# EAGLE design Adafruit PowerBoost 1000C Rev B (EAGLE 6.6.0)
COMPANY: ADAFRUIT INDUSTRIES; DRAWN: KTOWN; REV: A
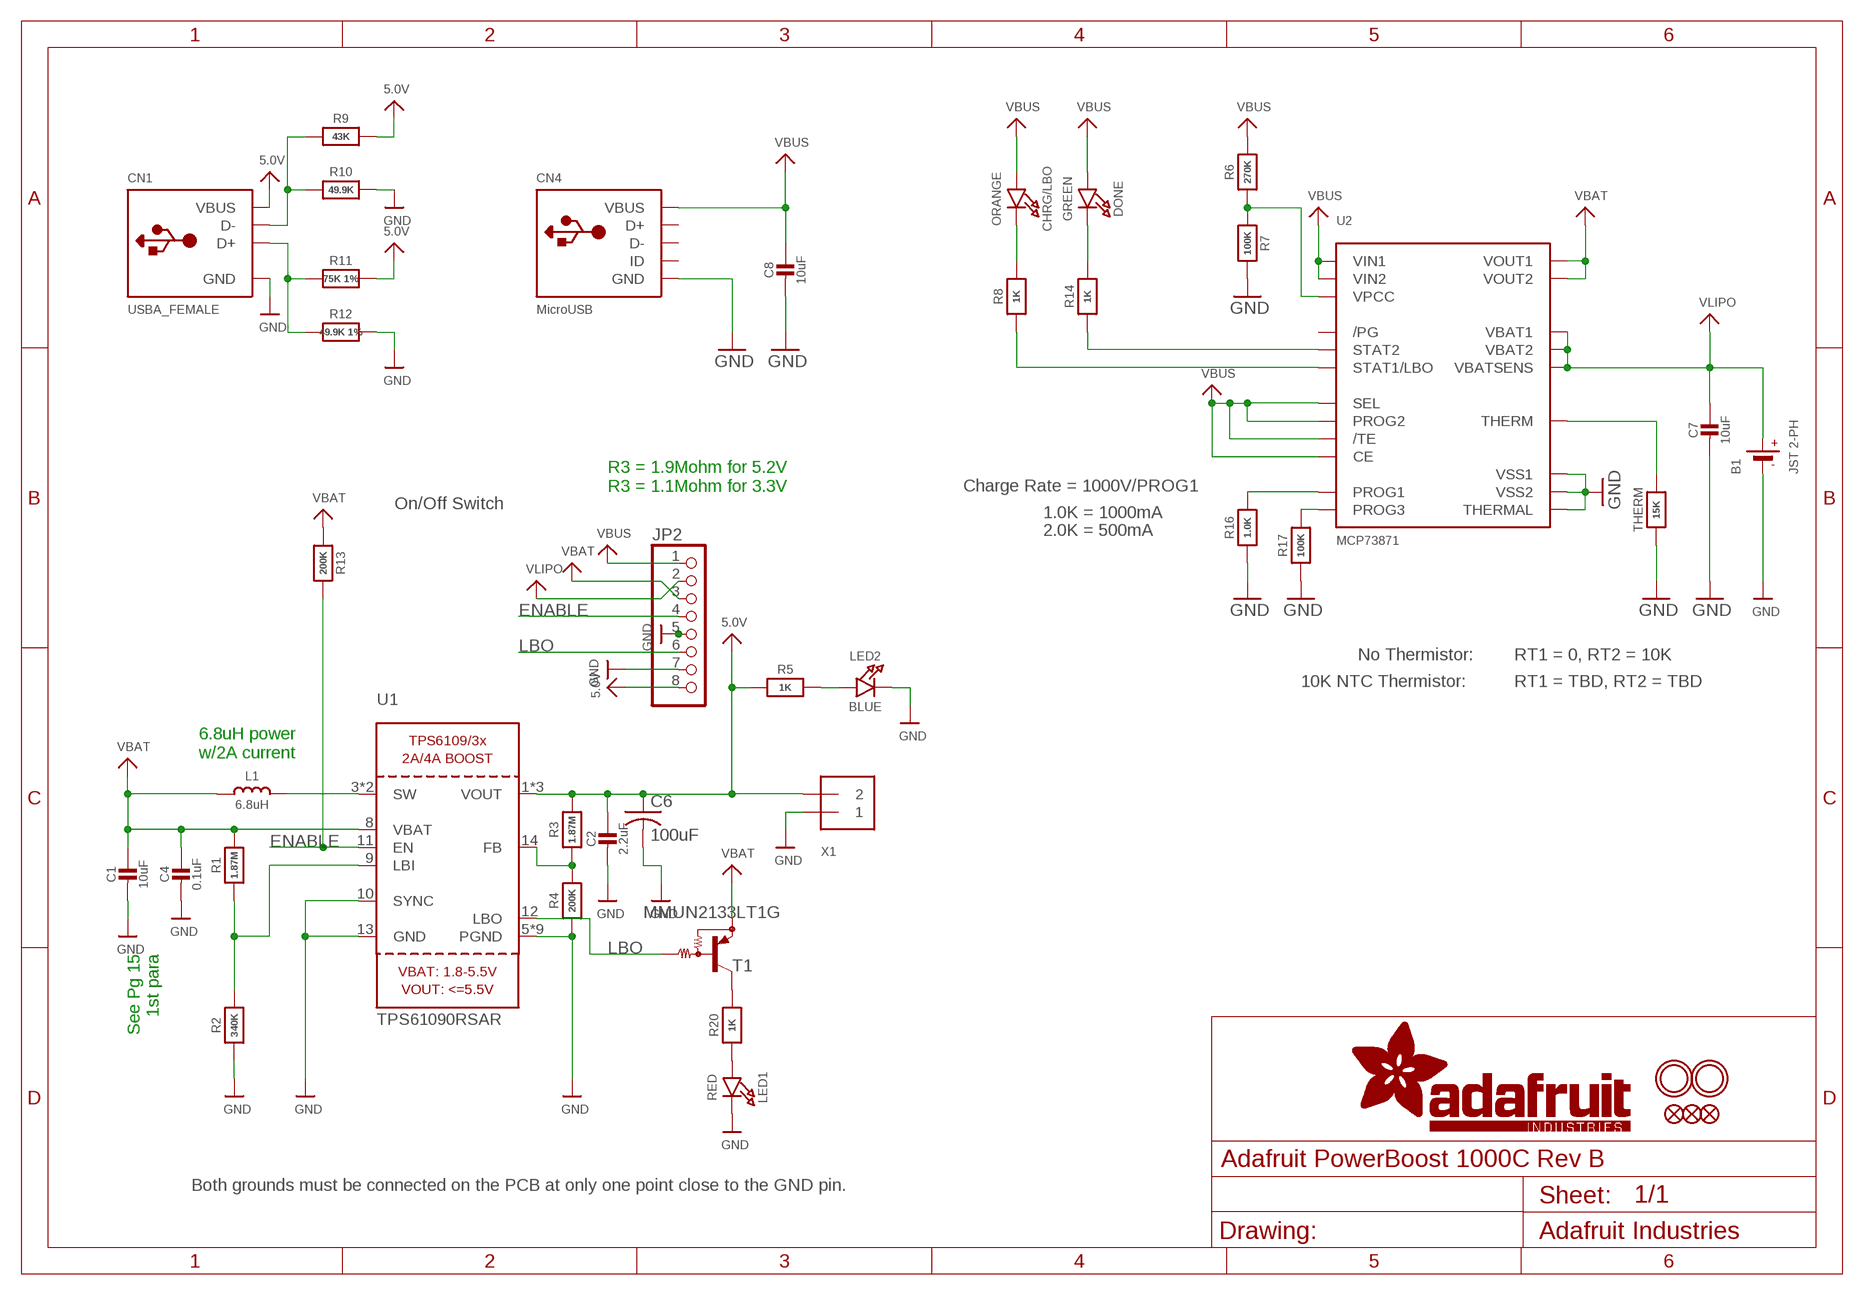
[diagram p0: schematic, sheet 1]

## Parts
B1  JST 2-PH  BATTERY  [JSTPH2]
C1  10uF  CAP_CERAMIC0805-NOOUTLINE  [0805-NO]
C2  2.2uF  CAP_CERAMIC0805-NOOUTLINE  [0805-NO]
C4  0.1uF  CAP_CERAMIC0805_10MGAP  [0805_10MGAP]
C6  100uF  C-USC1210  [C1210]
C7  10uF  CAP_CERAMIC0805-NOOUTLINE  [0805-NO]
C8  10uF  CAP_CERAMIC0805-NOOUTLINE  [0805-NO]
CHRG/LBO  ORANGE  LED0805_NOOUTLINE  [CHIPLED_0805_NOOUTLINE]
CN1  USBA_FEMALE  USB_TYPEAPTHFML  [USB_HOST-PTH]
CN4  MicroUSB  USBMICRO_20329  [4UCONN_20329]
DONE  GREEN  LED0805_NOOUTLINE  [CHIPLED_0805_NOOUTLINE]
FID1  FIDUCIAL""  [FIDUCIAL_1MM]
FID2  FIDUCIAL""  [FIDUCIAL_1MM]
FID3  FIDUCIAL""  [FIDUCIAL_1MM]
JP2  HEADER-1X8ROUND  [1X08_ROUND]
L1  6.8uH  INDUCTORTDK_VLC5045  [INDUCTOR_5X5MM_TDK_VLC5045]
LED1  RED  LED0805_NOOUTLINE  [CHIPLED_0805_NOOUTLINE]
LED2  BLUE  LED0805_NOOUTLINE  [CHIPLED_0805_NOOUTLINE]
R1  1.87M  RESISTOR_0805MP  [_0805MP]
R2  340K  RESISTOR_0805MP  [_0805MP]
R3  1.87M  RESISTOR0805_NOOUTLINE  [0805-NO]
R4  200K  RESISTOR0805_NOOUTLINE  [0805-NO]
R5  1K  RESISTOR0805_NOOUTLINE  [0805-NO]
R6  270K  RESISTOR0805_NOOUTLINE  [0805-NO]
R7  100K  RESISTOR0805_NOOUTLINE  [0805-NO]
R8  1K  RESISTOR0805_NOOUTLINE  [0805-NO]
R9  43K  RESISTOR0805_NOOUTLINE  [0805-NO]
R10  49.9K  RESISTOR0805_NOOUTLINE  [0805-NO]
R11  75K 1%  RESISTOR0805_NOOUTLINE  [0805-NO]
R12  49.9K 1%  RESISTOR0805_NOOUTLINE  [0805-NO]
R13  200K  RESISTOR0805_NOOUTLINE  [0805-NO]
R14  1K  RESISTOR0805_NOOUTLINE  [0805-NO]
R16  1.0K  RESISTOR0805_NOOUTLINE  [0805-NO]
R17  100K  RESISTOR0805_NOOUTLINE  [0805-NO]
R20  1K  RESISTOR0805_NOOUTLINE  [0805-NO]
T1  MMUN2133LT1G  MUN2114T1-PNP_DRIVER-SC59-BEC  [SC59-BEC]
THERM  15K  RESISTOR0805_NOOUTLINE  [0805-NO]
U1  TPS61090RSAR  VREG_TPS6103X  [PVQFN-16]
U2  MCP73871  [QFN20_4MM]
U$10  MOUNTINGHOLE2.5  [MOUNTINGHOLE_2.5_PLATED]
U$11  MOUNTINGHOLE2.5  [MOUNTINGHOLE_2.5_PLATED]
X1  TERMBLOCK_1X2  [TERMBLOCK_1X2-3.5MM]

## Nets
5.0V: C2.1 C6.1 CN1.VBUS JP2.8 R3.2 R5.1 R9.2 R11.2 U1.1(VOUT) U1.15(VOUT) U1.16(VOUT) X1.2
D+: CN1.D+ R11.1 R12.1
D-: CN1.D- R9.1 R10.1
ENABLE: JP2.4 R13.2 U1.11(EN)
GND: B1.1(-) C1.2 C2.2 C4.2 C6.2 C7.2 C8.2 CN1.GND CN4.BASE@1(GND) CN4.BASE@2(GND) CN4.GND CN4.SPRT@1(GND) CN4.SPRT@2(GND) CN4.SPRT@3(GND) CN4.SPRT@4(GND) JP2.5 JP2.7 LED1.C LED2.C R2.1 R4.1 R7.2 R10.2 R12.2 R16.1 R17.1 THERM.1 U1.5(PGND) U1.6(PGND) U1.7(PGND) U1.10(SYNC) U1.13(GND) U1.P$18(PGND) U1.P$19(PGND) U1.P$20(PGND) U1.P$21(PGND) U1.P$22(PGND) U1.THERMAL(PGND) U2.P$10(VSS1) U2.P$11(VSS2) U2.P$21(THERMAL) X1.1
LBO: JP2.6 T1.B U1.12(LBO)
N$1: L1.P$2 U1.3(SW) U1.4(SW)
N$2: LED1.A R20.1
N$3: R1.1 R2.2 U1.9(LBI)
N$4: LED2.A R5.2
N$5: R3.1 R4.2 U1.14(FB)
N$6: R20.2 T1.C
N$7: R6.1 R7.1 U2.P$2(VPCC)
N$8: DONE.C R14.2
N$9: R14.1 U2.P$7(STAT2)
N$10: THERM.2 U2.P$5(THERM)
N$11: R8.1 U2.P$8(STAT1/LBO)
N$12: CHRG/LBO.C R8.2
N$13: R17.2 U2.P$12(PROG3)
N$16: R16.2 U2.P$13(PROG1)
VBAT: C1.1 C4.1 JP2.3 L1.P$1 R1.2 R13.1 T1.E U1.8(VBAT) U2.P$1(VOUT1) U2.P$20(VOUT2)
VBUS: C8.1 CHRG/LBO.A CN4.VBUS DONE.A JP2.1 R6.2 U2.P$3(SEL) U2.P$4(PROG2) U2.P$9(/TE) U2.P$17(CE) U2.P$18(VIN1) U2.P$19(VIN2)
VLIPO: B1.2(+) C7.1 JP2.2 U2.P$14(VBAT1) U2.P$15(VBAT2) U2.P$16(VBATSENS)
Unconnected: CN4.D+ CN4.D- CN4.ID U2.P$6(/PG)

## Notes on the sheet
- R3 = 1.9Mohm for 5.2V
  R3 = 1.1Mohm for 3.3V
- Charge Rate = 1000V/PROG1
- On/Off Switch
- 1.0K = 1000mA
- 2.0K = 500mA
- No Thermistor: | RT1 = 0, RT2 = 10K
- 10K NTC Thermistor: | RT1 = TBD, RT2 = TBD
- 6.8uH power
  w/2A current
- See Pg 15
  1st para
- Both grounds must be connected on the PCB at only one point close to the GND pin.

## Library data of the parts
B1 = microbuilder:BATTERY: CR1220 SMT - Digikey: 3001K-ND
C1 C2 C4 C7 C8 = microbuilder:CAP_CERAMIC: Ceramic Capacitors
C6 = rcl:C-US: CAPACITOR, American symbol
CHRG/LBO DONE LED1 LED2 = microbuilder:LED: LED
CN1 = microbuilder:USB_TYPEA: USB - Type A Connectors Male types stick out and are inserted into a PC or matching females parts (these are the connectors used on USB Memory Sticks, etc.). Female parts are generally used for USB Host and accept a male-type connector. SMT - 4UCON: 10017 PTHFML - Digikey: 609-1045-ND, 4UCon: 05241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
CN4 = microbuilder:USB: USB Connectors USBMINIB - Surface Mount Female Mini-B USB Connector 4UConnector: 06564
FID1-FID3 = microbuilder:FIDUCIAL: Fiducial Alignment Points; BOM: EXCLUDE
JP2 = microbuilder:HEADER-1X8: PIN HEADER
L1 = microbuilder:INDUCTOR: Inductors
R1-R14 R16 R17 R20 THERM = microbuilder:RESISTOR: Resistors
T1 = transistor:*-PNP_DRIVER-: PNP Bias Resistor Transistor
U1 = microbuilder:VREG_TPS6103X: TPS6103x 4A Boost - 1.8-5.5V Input, Adjustable Output to 5.5V
U2 = microbuilder:MCP73871: MCP73871 Lithium Polymer Battery Charger Digikey: MCP73871-2CCI/ML-ND
U$10 U$11 = microbuilder:MOUNTINGHOLE: Mounting Hole; BOM: EXCLUDE
X1 = microbuilder:TERMBLOCK_1X2: 3.5mm Terminal block

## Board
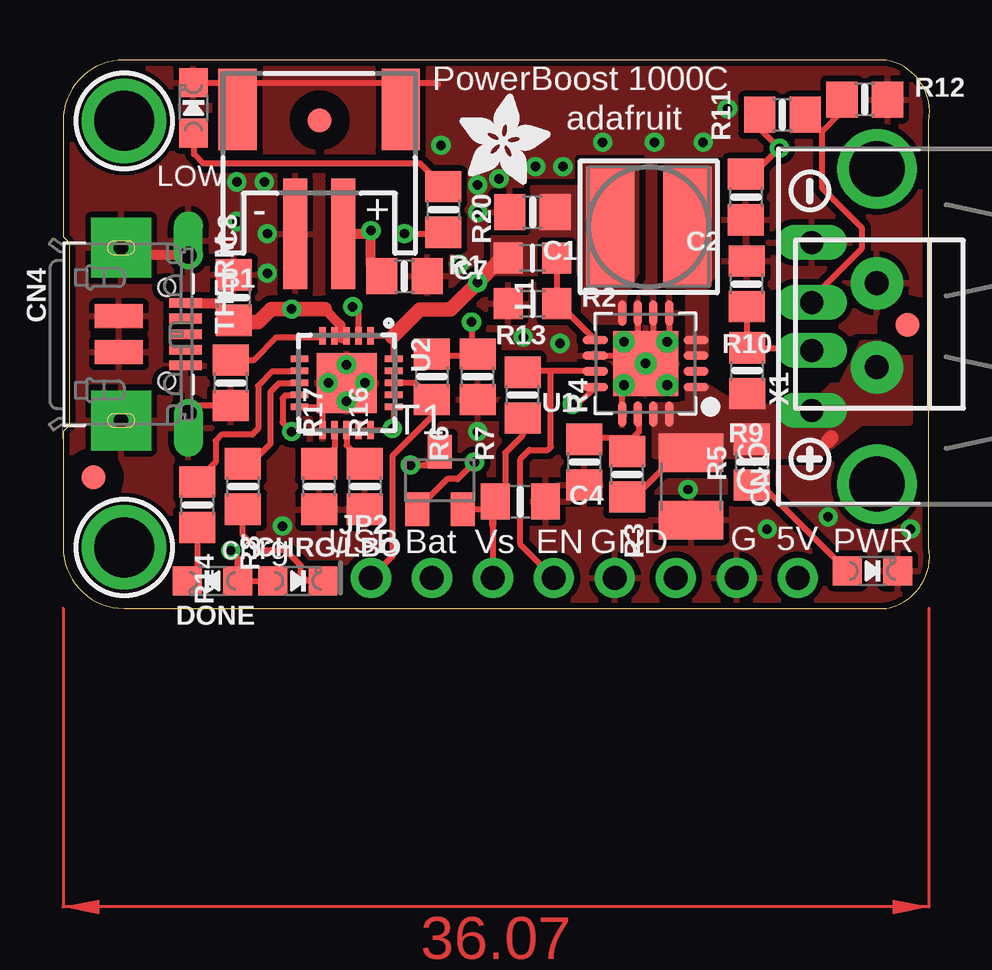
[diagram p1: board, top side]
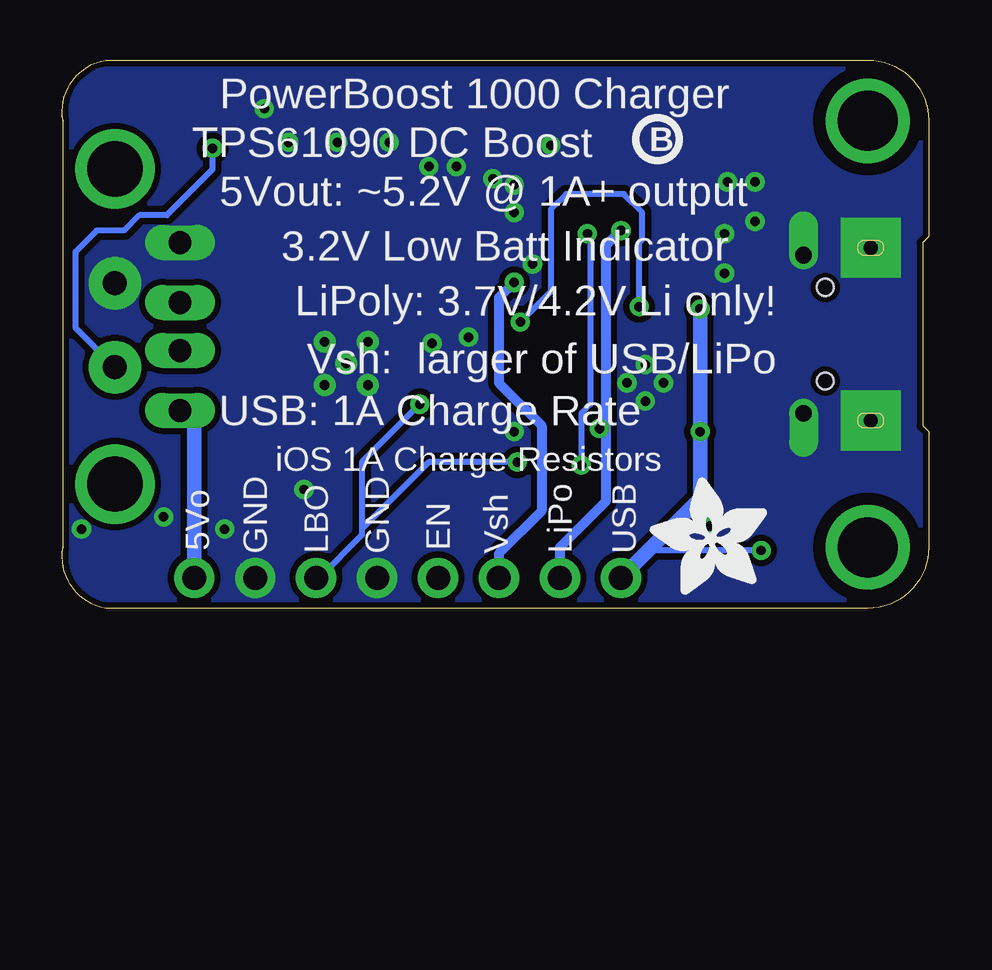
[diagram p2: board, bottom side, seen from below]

Size 36.1 x 22.86 mm. Coordinates in mm from the lower left corner, seen from the top.
Outline: 34.29,22.86 2.54,22.86 arc90 0,20.32 0,15.49 0.25,15.24 0.25,7.62 0,7.37 0,2.54 arc90 2.54,0 34.29,0 arc90 36.07,2.54 36.07,20.32 arc90 34.29,22.86
Copper layers (1*16): Top 0.035mm / dielectric 1.5mm / Bottom 0.035mm
Design rules "adafruit *": minimum track width 8mil, minimum drill 15.5mil, track to track 8mil, track to pad 8mil, pad to pad 8mil, via to via 8mil, smd to smd 8mil, copper to edge 10mil, drill to drill 8mil, minimum pad ring 10mil, minimum via ring 8mil, stop-mask expansion 2mil, vias tented up to drill 20mil, thermal gap 10mil
tRestrict: area 22.9,7.9 to 23.1,8.3; area 24.9,12.1 to 25,12.4; area 24.3,12.1 to 24.4,12.4

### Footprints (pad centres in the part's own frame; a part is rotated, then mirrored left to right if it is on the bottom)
JSTPH2 = smd 1 x 4.6: 1 -1,-3.7; 2 1,-3.7 | smd 1.6 x 3.4: NC1 -3.4,1.5; NC2 3.4,1.5
0805-NO = smd 1.3 x 1.5: 1 -0.95,0; 2 0.95,0
0805_10MGAP = smd 1.2 x 1.5: 1 -1.05,0; 2 1.05,0
C1210 = smd 1.6 x 2.7: 1 -1.4,0; 2 1.4,0
CHIPLED_0805_NOOUTLINE = smd 1.2 x 1.2: A 0,-1.05; C 0,1.05
USB_HOST-PTH = drill 0.95 long: D+ 1,6.52; D- -1,6.52; GND 3.5,6.52; VBUS -3.5,6.52 | drill 2.3 pad 2.9: S1 -6.57,3.81; S2 6.57,3.81
4UCONN_20329 = smd 1 x 2: BASE@1 -0.75,-2; BASE@2 0.75,-2 | smd 0.4 x 1.35: D+ 0,0.775; D- -0.65,0.775; GND 1.3,0.775; ID 0.65,0.775; VBUS -1.3,0.775 | drill 0.7 offset: SPRT@1 -3.3,0.9; SPRT@2 3.3,0.9 | drill 0.6 pad 2.5 square: SPRT@3 -3.6,-1.9; SPRT@4 3.6,-1.9 | hole 0.7: -1.95,0; 1.95,0
FIDUCIAL_1MM = smd 1 x 1: 1 0,0
1X08_ROUND = drill 1 pad 1.676: 1 -8.89,0; 2 -6.35,0; 3 -3.81,0; 4 -1.27,0; 5 1.27,0; 6 3.81,0; 7 6.35,0; 8 8.89,0
INDUCTOR_5X5MM_TDK_VLC5045 = smd 2 x 5: P$1 -1.6,0; P$2 1.6,0
_0805MP = smd 1.2 x 1.3: 1 -1.016,0; 2 1.016,0
SC59-BEC = smd 1 x 1.4: B -0.95,-1.2; C 0,1.2; E 0.95,-1.2
PVQFN-16 = smd 1.05 x 0.35: 1 -2.1,0.975; 2 -2.1,0.325; 3 -2.1,-0.325; 4 -2.1,-0.975; 9 2.1,-0.975; 10 2.1,-0.325; 11 2.1,0.325; 12 2.1,0.975 | smd 0.35 x 1.05: 5 -0.975,-2.1; 6 -0.325,-2.1; 7 0.325,-2.1; 8 0.975,-2.1; 13 0.975,2.1; 14 0.325,2.1; 15 -0.325,2.1; 16 -0.975,2.1 | drill 0.4: P$18 0,0; P$19 -0.9,0.9; P$20 0.9,0.9; P$21 0.9,-0.9; P$22 -0.9,-0.9 | smd 2.7 x 2.7: THERMAL 0,0
QFN20_4MM = smd 0.73 x 0.28: P$1 -1.965,1; P$2 -1.965,0.5; P$3 -1.965,0; P$4 -1.965,-0.5; P$5 -1.965,-1; P$11 1.965,-1; P$12 1.965,-0.5; P$13 1.965,0; P$14 1.965,0.5; P$15 1.965,1 | smd 0.28 x 0.73: P$6 -1,-1.965; P$7 -0.5,-1.965; P$8 0,-1.965; P$9 0.5,-1.965; P$10 1,-1.965; P$16 1,1.965; P$17 0.5,1.965; P$18 0,1.965; P$19 -0.5,1.965; P$20 -1,1.965 | smd 2.5 x 2.5: P$21 0,0
MOUNTINGHOLE_2.5_PLATED = drill 2.5 pad 3.2: P$1 0,0
TERMBLOCK_1X2-3.5MM = drill 1 pad 2.184: 1 1.8,0; 2 -1.7,0

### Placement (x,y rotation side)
B1  10.67,19.3 0 top
C1  19.56,16.51 180 top
C2  28.45,17.14 270 top
C4  19.05,4.45 0 top
C6  26.16,5.08 270 top
C7  14.22,13.84 0 top
C8  7.11,12.95 90 top
CHRG/LBO  9.78,1.14 270 top
CN1  37.72,11.75 90 top
CN4  4.32,11.43 270 top
DONE  6.22,1.14 90 top
FID1  35.18,11.81 0 top
FID2  10.69,20.34 90 top
FID3  1.27,5.46 0 top
JP2  21.72,1.27 0 top
L1  24.4,15.9 0 top
LED1  5.43,20.86 0 top
LED2  33.72,1.56 270 top
R1  19.56,14.61 180 top
R2  19.56,12.7 0 top
R3  23.5,5.59 270 top
R4  21.72,6.1 90 top
R5  28.7,6.1 270 top
R6  15.37,9.65 270 top
R7  17.27,9.65 270 top
R8  7.49,5.08 270 top
R9  28.5,9.91 270 top
R10  28.48,13.52 90 top
R11  29.97,20.57 180 top
R12  33.4,21.21 0 top
R13  19.14,8.89 90 top
R14  5.59,4.32 270 top
R16  12.57,5.08 90 top
R17  10.67,5.08 90 top
R20  15.84,16.62 270 top
T1  15.7,5.33 0 top
THERM  6.99,9.4 90 top
U1  24.27,10.21 180 top
U2  11.81,9.4 270 top
U$10  2.54,20.32 0 top
U$11  2.54,2.54 0 top
U$12  [PCBFEAT-REV-040]  11.3,19.56 0 bottom
U$25  [SYMBOL_PLUS]  31.11,6.22 0 top
U$26  [SYMBOL_MINUS]  31.11,17.4 90 top
U$28  [ADAFRUIT_5MM]  6.75,0.58 90 bottom
U$45  [ADAFRUIT_3.5MM]  16.51,17.65 0 top
X1  33.91,11.75 90 top

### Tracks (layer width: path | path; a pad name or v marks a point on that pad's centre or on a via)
5.0V  (via drill 0.39)
  Top 0.254: 32.38,8.38 32.13,8.38 32,8.25 CN1.VBUS | R11.2 29.02,20 v29.84,19.18 28.76,18.09 C2.1 | R3.2 23.82,4.64 25.02,5.84 25.52,5.84 C6.1
  Top 0.61: 31.88,6.99 32,7.11
  Bottom 0.254: v29.84,19.18 29.84,18.29 31.75,16.38 32.89,16.38 33.53,15.75 34.67,15.75 35.56,14.86 35.56,11.7 X1.2
  Bottom 0.61: JP2.8 30.61,7.66 CN1.VBUS
  pour Top (isolate 0.254, no thermals): 24.64,8.51 24.64,6.35 31.5,6.35 33.27,7.75 35.31,7.75 35.31,11.05 33.27,11.05 32.38,9.27 32,9.27 31.11,8.38 28.19,8.38 26.8,9.27 26.04,9.27 26.04,8.51
D+
  Top 0.254: CN1.D+ 31.2,12.91 33.27,14.99 33.27,15.88 31.62,17.53 31.62,19.87 | 31.62,19.87 R11.1 | R12.1 32.45,20.7 31.62,19.87
D-
  Top 0.254: R10.1 28.48,10.88 R9.1 31.09,10.86 CN1.D-
ENABLE
  Top 0.254: U1.11 20.32,9.88 | 20.32,9.88 19.19,9.88 R13.2 | JP2.4 19.05,2.67 19.05,6.22 19.43,6.6 20.19,6.6 20.32,6.73 20.32,9.88
GND  (via drill 0.39)
  Top 0.254: U1.13 23.3,9.07 23.5,9.27 23.41,9.27 U1.P$20 | U1.10 23.61,10.53 23.62,10.54 23.37,10.79 U1.P$21 23.44,11.18 23.88,11.18 23.95,11.25 U1.7 | U1.6 24.6,10.96 24.77,10.79 | U1.5 25.25,11.18 U1.P$22 | THERM.1 5.54,8.45 CN4.SPRT@2 5.22,8.26 5.33,8.26 | LED1.C 15.55,21.91 15.62,21.84 | U2.P$11 10.81,9.16 v11.05,9.4 | U2.P$10 11.57,8.4 v11.81,8.64
  Top 0.406: CN4.SPRT@1 2.85,14.73 | 4.91,7.83 5.33,8.26
  other vias: 27.69,20.83 26.04,4.95 29.34,3.3 31.88,3.81 35.31,3.3 19.18,11.3 17.27,7.37 11.81,10.16 9.14,3.43 20.7,11.05 12.57,9.4 16.51,14.35 19.68,18.41 20.83,18.41 15.75,19.3 17.27,16.51 18.16,17.91 17.27,17.65 8.51,15.62 8.51,13.97 8.38,17.78 7.24,17.78 7.24,16.13 26.67,19.43 24.64,19.43 22.48,19.43
  pour Top (isolate 0.254, rank 2): 0,-0.13 0,22.61 36.07,22.73 36.07,0
  pour Bottom (isolate 0.254, no thermals): 0,22.73 36.07,22.99 36.07,0.25 0,0
LBO  (via drill 0.39)
  Top 0.254: U1.12 21.45,8.51 v21.21,8.51 | v17.14,6.1 16.44,5.39 16,5.39 T1.B
  Bottom 0.254: v21.21,8.51 23.62,6.1 23.62,3.3 | 23.62,3.3 23.62,3.05 25.4,1.27 JP2.6 | v17.14,6.1 20.83,6.1 23.62,3.3
N$1
  pour Top (isolate 0.254, no thermals): 26.04,10.54 26.8,10.54 26.8,13.46 27.05,13.84 27.05,18.41 25.15,18.41 25.15,13.46 26.04,13.46
N$2
  Top 0.254: R20.1 14.87,18.54 5.84,18.54 5.46,18.92 5.46,19.78 LED1.A
N$3
  Top 0.254: R1.1 R2.2 20.94,12.34 21.02,12.34 U1.9
N$4
  Top 0.254: R5.2 29.08,5.15 LED2.A
N$5
  Top 0.254: 23.75,7.11 24,7.37 24,8.05 U1.14 | R4.2 21.72,7.11 23.75,7.11 | R3.1 23.5,6.86 23.75,7.11
N$6  (via drill 0.39)
  Top 0.254: v14.48,5.97 15.13,5.97 T1.C | v14.22,15.62 15.79,15.62 R20.2
  Bottom 0.254: v14.22,15.62 14.1,15.49 14.1,8.51 14.48,8.13 v14.48,5.97
N$7  (via drill 0.39)
  Top 0.254: R6.1 15.43,10.6 15.49,10.54 17.21,10.54 R7.1 | R7.1 17.33,10.54 | U2.P$2 12.31,12.33 v12.06,12.57 | v17.02,11.94 17.02,10.86 R7.1
  Bottom 0.254: v12.06,12.57 12.06,15.24 11.94,15.37 11.94,16.51 12.7,17.27 15.11,17.27 15.75,16.64 15.75,13.21 v17.02,11.94
N$8
  Top 0.254: R14.2 5.59,1.56 DONE.C
N$9
  Top 0.254: R14.1 5.59,5.33 6.35,6.1 6.35,6.99 6.6,7.24 7.87,7.24 8.13,7.49 8.13,9.27 8.74,9.88 9.83,9.88 U2.P$7
N$10
  Top 0.254: THERM.2 7.93,10.35 8.89,11.3 10.82,11.3 U2.P$5
N$11
  Top 0.254: R8.1 7.69,6.22 8,6.22 8.64,6.86 8.64,9.02 9,9.38 9.83,9.38 U2.P$8
N$12
  Top 0.254: CHRG/LBO.C 10.16,1.14 9.91,1.4 9.91,1.78 9.27,2.41 8.13,2.41 7.49,3.05 R8.2
N$13
  Top 0.254: U2.P$12 11.31,6.67 R17.2
N$16
  Top 0.254: U2.P$13 11.81,6.79 R16.2
VBAT  (via drill 0.39)
  Top 0.254: R13.1 19.14,7.21 18.41,6.48 18.41,4.86 C4.1 17.69,4.13 T1.E | 17.91,3.49 JP2.3 | U2.P$1 13.66,11.36 13.72,11.3 13.83,11.19 13.78,11.14 U2.P$20
  Top 0.305: 17.91,3.49 17.91,4.35 C4.1
  Top 0.61: 13.72,11.3 14.86,12.45 16.13,12.45 v17.27,13.59 18.16,14.48 18.54,14.48 R1.2
  Bottom 0.406: v17.27,13.59 17.91,12.95 17.91,9.4 16.13,7.62 16.13,4.06 17.91,2.29 JP2.3
  pour Top (isolate 0.254, no thermals): 23.37,11.94 21.72,11.94 21.72,18.54 23.88,18.54 23.88,13.97 23.37,12.95
  pour Top (no thermals): 19.56,17.53 19.56,15.49 17.91,15.49 17.91,13.97 21.59,13.97 21.72,17.53
VBUS  (via drill 0.39)
  Top 0.254: v9.53,7.37 9.14,7.75 9.14,8.76 9.27,8.88 9.83,8.88 U2.P$9 | CHRG/LBO.A DONE.A 7.27,2.12 v6.99,2.41 | JP2.1 13.72,2.16 13.72,6.35 15.37,8 R6.2 14.68,9.38 13.79,9.38 U2.P$18 | U2.P$4 U2.P$3 11.64,11.36 11.63,11.35 | U2.P$19 U2.P$18 | U2.P$18 U2.P$17
  Top 0.406: CN4.VBUS 6.39,12.73 C8.1 | 10.89,12.48 11.56,11.81 11.56,11.43 | 15.18,8.88 R6.2
  Top 0.61: 10.89,12.48 v9.53,12.48 8.67,12.48 8.13,11.94 7.18,11.94 C8.1 | 11.63,11.35 11.56,11.43
  Bottom 0.254: v6.99,2.41 11.68,2.41
  Bottom 0.61: v9.53,12.48 v9.53,7.37 9.53,4.57 11.68,2.41 JP2.1
VLIPO  (via drill 0.39)
  Top 0.254: U2.P$14 U2.P$15 13.66,7.43 v13.72,7.49 13.78,7.55 U2.P$16
  Top 0.406: B1.2 12.68,15.6 v12.83,15.75 12.83,14.29 C7.1
  Bottom 0.406: v13.72,7.49 13.46,7.49 | JP2.2 15.37,2.54 13.46,4.45 13.46,7.49 | v12.83,15.75 13.46,15.11 13.46,7.49
(copper drawn outside any net)
  shapes: Top area x1

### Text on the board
tPlace: PowerBoost 1000C | adafruit | LOW | - | + | PWR | chrg | USB | Bat | Vs | EN | GND | G | 5V
bPlace: PowerBoost 1000 Charger | TPS61090 DC Boost | 5Vout: ~5.2V @ 1A+ output | 3.2V Low Batt Indicator | LiPoly: 3.7V/4.2V Li only! | Vsh: larger of USB/LiPo | USB: 1A Charge Rate | iOS 1A Charge Resistors | USB | LiPo | Vsh | EN | GND | LBO | GND | 5Vo

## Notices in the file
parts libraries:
microbuilder: This work is placed in the public domain, and may be freely used for commercial and non-commercial work with the following conditions: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
